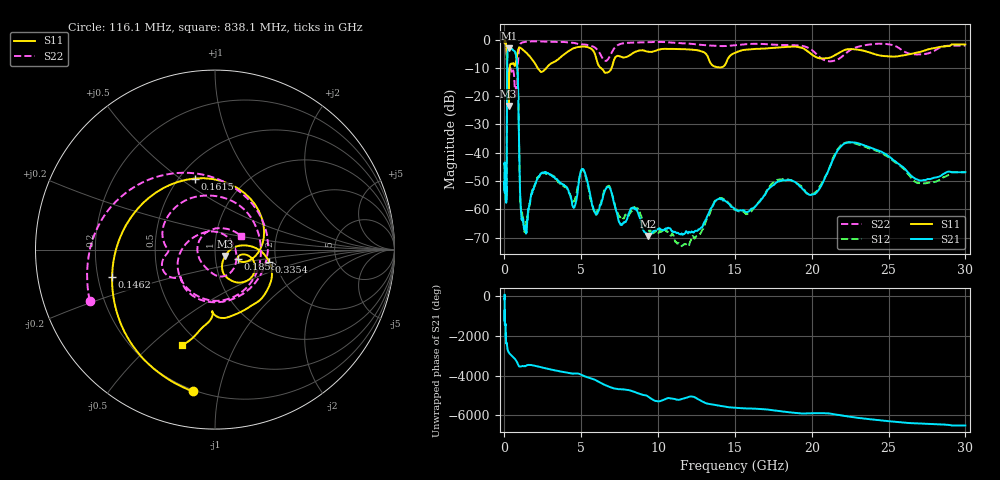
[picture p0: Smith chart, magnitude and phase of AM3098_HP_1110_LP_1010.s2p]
! Date/Time: Thu, Feb 28, 2019 8:46 AM
! Network Analyzer: Agilent Technologies E8364B Rev: A.07.50.67
! Sweep from 0.010 to 30.000 GHz, 1601 Points, Sweep Type: LOG
! Power Supply: 5.023 V, 0.002 A
# Hz S DB R 50
!freq MagS11 AngS11 MagS21 AngS21 MagS12 AngS12 MagS22 AngS22
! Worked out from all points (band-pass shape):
!   1601 points, 10 MHz to 30 GHz, reference 50 ohm
!   highest |S21| = -3.09 dB at 291.6 MHz (marker M1); lowest = -69.4 dB at 9.349 GHz (marker M2)
!   |S21| within 3 dB of the highest: 183.7 MHz to 772.6 MHz (588.8 MHz wide, 123 % of centre)
!   lowest |S11| = -23.5 dB at 265.1 MHz (marker M3), VSWR 1.14, Z = 55.9 - j3.98 ohm
!   |S11| at or under -10 dB: 169.7 MHz to 338.7 MHz (169 MHz wide, 66.5 % of centre); 2.156 GHz to 2.735 GHz (579.1 MHz wide, 23.7 % of centre); 6.267 GHz to 6.975 GHz (708.2 MHz wide, 10.7 % of centre)
!   |S22| runs from -20.2 to -0.6 dB; largest |S21 - S12| = 0.012
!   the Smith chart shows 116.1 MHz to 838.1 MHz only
!   S11 on the Smith chart (normalised r, x): 116.1 MHz: 0.19, -0.84; 146.2 MHz: 0.26, -0.12; 161.5 MHz: 0.60, +0.57; 185.8 MHz: 1.28, -0.14; 335.4 MHz: 1.84, -0.28; 838.1 MHz: 0.41, -0.63
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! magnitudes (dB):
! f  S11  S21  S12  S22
! 10 MHz  -0.4  -44.0  -44.6  -0.6
! 38.04 MHz  -0.3  -50.7  -50.1  -0.8
! 116.1 MHz  -2.0  -57.2  -54.3  -2.5
! 144.7 MHz  -4.3  -50.2  -50.6  -5.5
! 146.2 MHz  -4.5  -49.1  -48.9  -5.8
! 161.5 MHz  -7.7  -23.4  -23.5  -10.5
! 185.8 MHz  -17.3  -5.7  -5.7  -12.2
! 265.1 MHz  -23.5  -3.2  -3.1  -11.7
! 291.6 MHz  -16.3  -3.1  -3.0  -11.3
! 335.4 MHz  -10.2  -3.2  -3.1  -10.0
! 550.5 MHz  -8.4  -3.7  -3.6  -10.9
! 838.1 MHz  -5.0  -9.9  -9.8  -15.6
! 1.109 GHz  -3.1  -63.4  -61.1  -1.1
! 2.084 GHz  -9.3  -49.8  -49.7  -0.6
! 4.525 GHz  -3.0  -59.5  -57.1  -1.2
! 5.128 GHz  -2.4  -45.8  -46.3  -1.7
! 7.926 GHz  -6.1  -64.0  -62.5  -1.1
! 9.349 GHz  -4.3  -69.4  -66.8  -0.9
! 11.95 GHz  -3.5  -68.5  -72.7  -1.4
! 20.1 GHz  -5.6  -54.7  -54.6  -4.1
! 22.67 GHz  -3.4  -36.3  -36.5  -3.2
! 30 GHz  -1.7  -46.9  -46.8  -2.1
